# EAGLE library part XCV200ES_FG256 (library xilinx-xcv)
xcv200es_fg256 edit this description Auto generated by make-symbol-device-package-bsdl.ulp Rev. 26 Source: xcv200es_fg256.bsd
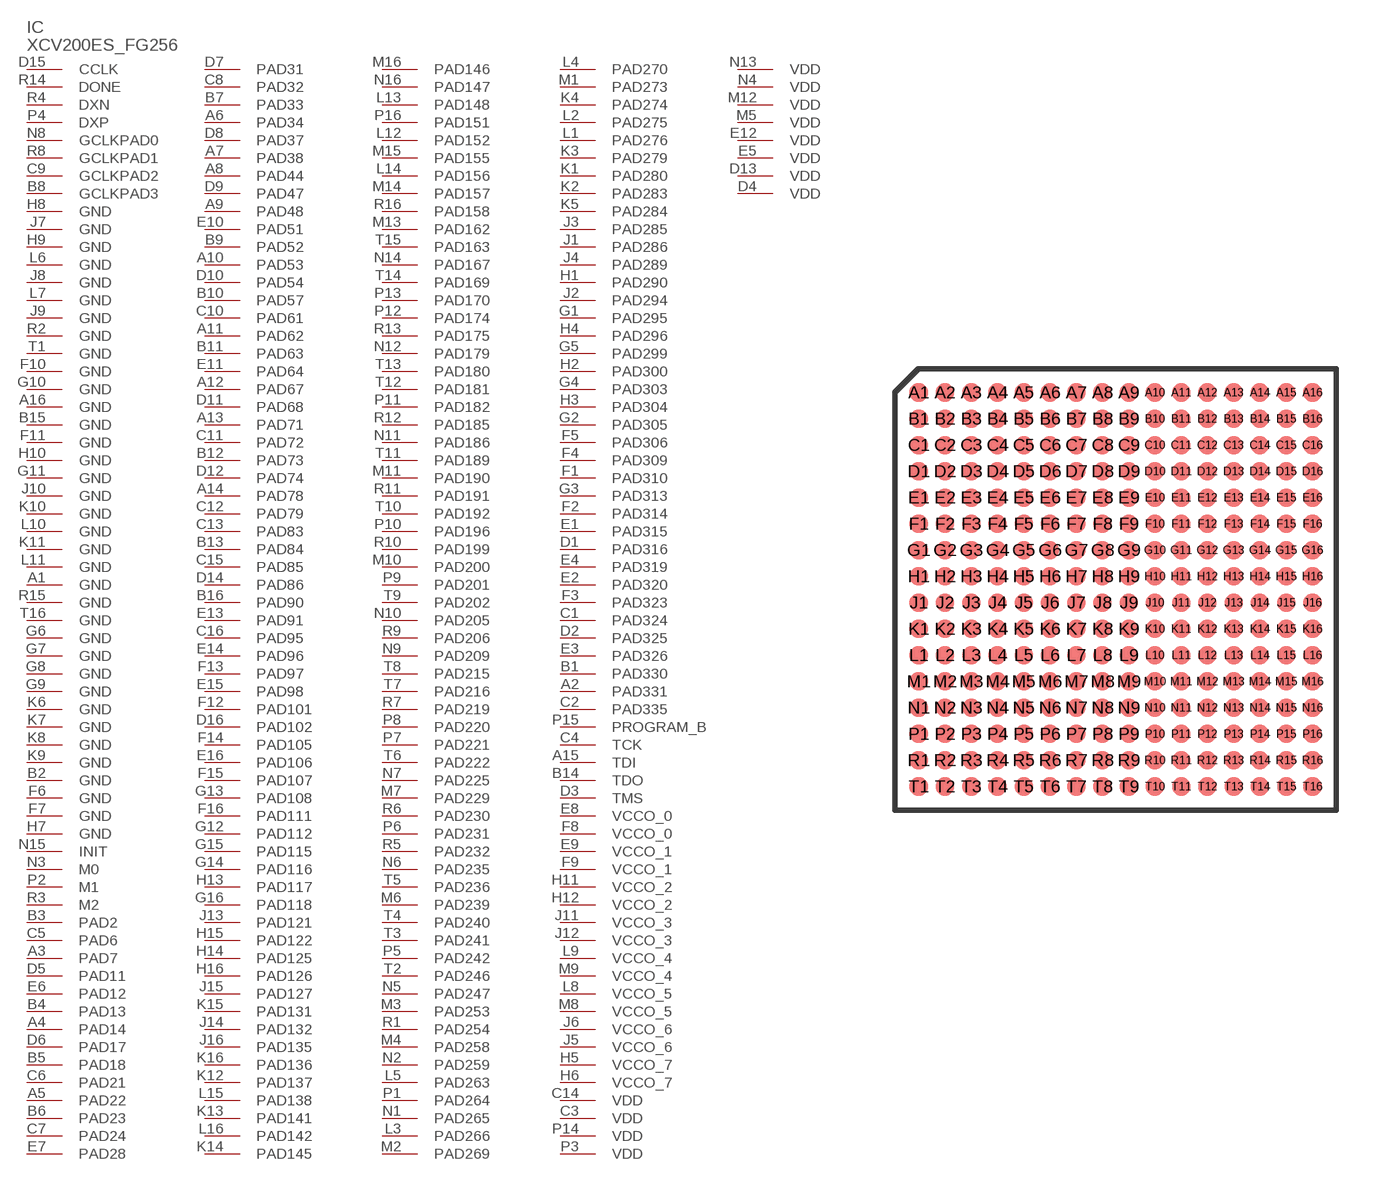
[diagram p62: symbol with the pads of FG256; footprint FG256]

Designator prefix IC

## XCV200ES_FG256 (OC_FARNELL: unknown; OC_NEWARK: unknown)  [FG256]
A1  GND  pwr
A2  PAD331
A3  PAD7
A4  PAD14
A5  PAD22
A6  PAD34
A7  PAD38
A8  PAD44
A9  PAD48
A10  PAD53
A11  PAD62
A12  PAD67
A13  PAD71
A14  PAD78
A15  TDI  in
A16  GND  pwr
B1  PAD330
B2  GND  pwr
B3  PAD2
B4  PAD13
B5  PAD18
B6  PAD23
B7  PAD33
B8  GCLKPAD3  in
B9  PAD52
B10  PAD57
B11  PAD63
B12  PAD73
B13  PAD84
B14  TDO  out
B15  GND  pwr
B16  PAD90
C1  PAD324
C2  PAD335
C3  VDD  pwr
C4  TCK  in
C5  PAD6
C6  PAD21
C7  PAD24
C8  PAD32
C9  GCLKPAD2  in
C10  PAD61
C11  PAD72
C12  PAD79
C13  PAD83
C14  VDD  pwr
C15  PAD85
C16  PAD95
D1  PAD316
D2  PAD325
D3  TMS  in
D4  VDD  pwr
D5  PAD11
D6  PAD17
D7  PAD31
D8  PAD37
D9  PAD47
D10  PAD54
D11  PAD68
D12  PAD74
D13  VDD  pwr
D14  PAD86
D15  CCLK
D16  PAD102
E1  PAD315
E2  PAD320
E3  PAD326
E4  PAD319
E5  VDD  pwr
E6  PAD12
E7  PAD28
E8  VCCO_0  pwr
E9  VCCO_1  pwr
E10  PAD51
E11  PAD64
E12  VDD  pwr
E13  PAD91
E14  PAD96
E15  PAD98
E16  PAD106
F1  PAD310
F2  PAD314
F3  PAD323
F4  PAD309
F5  PAD306
F6  GND  pwr
F7  GND  pwr
F8  VCCO_0  pwr
F9  VCCO_1  pwr
F10  GND  pwr
F11  GND  pwr
F12  PAD101
F13  PAD97
F14  PAD105
F15  PAD107
F16  PAD111
G1  PAD295
G2  PAD305
G3  PAD313
G4  PAD303
G5  PAD299
G6  GND  pwr
G7  GND  pwr
G8  GND  pwr
G9  GND  pwr
G10  GND  pwr
G11  GND  pwr
G12  PAD112
G13  PAD108
G14  PAD116
G15  PAD115
G16  PAD118
H1  PAD290
H2  PAD300
H3  PAD304
H4  PAD296
H5  VCCO_7  pwr
H6  VCCO_7  pwr
H7  GND  pwr
H8  GND  pwr
H9  GND  pwr
H10  GND  pwr
H11  VCCO_2  pwr
H12  VCCO_2  pwr
H13  PAD117
H14  PAD125
H15  PAD122
H16  PAD126
J1  PAD286
J2  PAD294
J3  PAD285
J4  PAD289
J5  VCCO_6  pwr
J6  VCCO_6  pwr
J7  GND  pwr
J8  GND  pwr
J9  GND  pwr
J10  GND  pwr
J11  VCCO_3  pwr
J12  VCCO_3  pwr
J13  PAD121
J14  PAD132
J15  PAD127
J16  PAD135
K1  PAD280
K2  PAD283
K3  PAD279
K4  PAD274
K5  PAD284
K6  GND  pwr
K7  GND  pwr
K8  GND  pwr
K9  GND  pwr
K10  GND  pwr
K11  GND  pwr
K12  PAD137
K13  PAD141
K14  PAD145
K15  PAD131
K16  PAD136
L1  PAD276
L2  PAD275
L3  PAD266
L4  PAD270
L5  PAD263
L6  GND  pwr
L7  GND  pwr
L8  VCCO_5  pwr
L9  VCCO_4  pwr
L10  GND  pwr
L11  GND  pwr
L12  PAD152
L13  PAD148
L14  PAD156
L15  PAD138
L16  PAD142
M1  PAD273
M2  PAD269
M3  PAD253
M4  PAD258
M5  VDD  pwr
M6  PAD239
M7  PAD229
M8  VCCO_5  pwr
M9  VCCO_4  pwr
M10  PAD200
M11  PAD190
M12  VDD  pwr
M13  PAD162
M14  PAD157
M15  PAD155
M16  PAD146
N1  PAD265
N2  PAD259
N3  M0  in
N4  VDD  pwr
N5  PAD247
N6  PAD235
N7  PAD225
N8  GCLKPAD0  in
N9  PAD209
N10  PAD205
N11  PAD186
N12  PAD179
N13  VDD  pwr
N14  PAD167
N15  INIT
N16  PAD147
P1  PAD264
P2  M1  in
P3  VDD  pwr
P4  DXP  pas
P5  PAD242
P6  PAD231
P7  PAD221
P8  PAD220
P9  PAD201
P10  PAD196
P11  PAD182
P12  PAD174
P13  PAD170
P14  VDD  pwr
P15  PROGRAM_B  in
P16  PAD151
R1  PAD254
R2  GND  pwr
R3  M2  in
R4  DXN  pas
R5  PAD232
R6  PAD230
R7  PAD219
R8  GCLKPAD1  in
R9  PAD206
R10  PAD199
R11  PAD191
R12  PAD185
R13  PAD175
R14  DONE
R15  GND  pwr
R16  PAD158
T1  GND  pwr
T2  PAD246
T3  PAD241
T4  PAD240
T5  PAD236
T6  PAD222
T7  PAD216
T8  PAD215
T9  PAD202
T10  PAD192
T11  PAD189
T12  PAD181
T13  PAD180
T14  PAD169
T15  PAD163
T16  GND  pwr

## Footprint FG256 (pad centres in mm)
Fine Pitch BGA (FG256) Auto generated by make-symbol-device-package-bsdl.ulp Rev. 26 Source: xcv100_fg256.bsd; fg256.pdf
smd 0.7 x 0.7: A1 -7.5,7.5; A2 -6.5,7.5; A3 -5.5,7.5; A4 -4.5,7.5; A5 -3.5,7.5; A6 -2.5,7.5; A7 -1.5,7.5; A8 -0.5,7.5; A9 0.5,7.5; A10 1.5,7.5; A11 2.5,7.5; A12 3.5,7.5; A13 4.5,7.5; A14 5.5,7.5; A15 6.5,7.5; A16 7.5,7.5; B1 -7.5,6.5; B2 -6.5,6.5; B3 -5.5,6.5; B4 -4.5,6.5; B5 -3.5,6.5; B6 -2.5,6.5; B7 -1.5,6.5; B8 -0.5,6.5; B9 0.5,6.5; B10 1.5,6.5; B11 2.5,6.5; B12 3.5,6.5; B13 4.5,6.5; B14 5.5,6.5; B15 6.5,6.5; B16 7.5,6.5; C1 -7.5,5.5; C2 -6.5,5.5; C3 -5.5,5.5; C4 -4.5,5.5; C5 -3.5,5.5; C6 -2.5,5.5; C7 -1.5,5.5; C8 -0.5,5.5; C9 0.5,5.5; C10 1.5,5.5; C11 2.5,5.5; C12 3.5,5.5; C13 4.5,5.5; C14 5.5,5.5; C15 6.5,5.5; C16 7.5,5.5; D1 -7.5,4.5; D2 -6.5,4.5; D3 -5.5,4.5; D4 -4.5,4.5; D5 -3.5,4.5; D6 -2.5,4.5; D7 -1.5,4.5; D8 -0.5,4.5; D9 0.5,4.5; D10 1.5,4.5; D11 2.5,4.5; D12 3.5,4.5; D13 4.5,4.5; D14 5.5,4.5; D15 6.5,4.5; D16 7.5,4.5; E1 -7.5,3.5; E2 -6.5,3.5; E3 -5.5,3.5; E4 -4.5,3.5; E5 -3.5,3.5; E6 -2.5,3.5; E7 -1.5,3.5; E8 -0.5,3.5; E9 0.5,3.5; E10 1.5,3.5; E11 2.5,3.5; E12 3.5,3.5; E13 4.5,3.5; E14 5.5,3.5; E15 6.5,3.5; E16 7.5,3.5; F1 -7.5,2.5; F2 -6.5,2.5; F3 -5.5,2.5; F4 -4.5,2.5; F5 -3.5,2.5; F6 -2.5,2.5; F7 -1.5,2.5; F8 -0.5,2.5; F9 0.5,2.5; F10 1.5,2.5; F11 2.5,2.5; F12 3.5,2.5; F13 4.5,2.5; F14 5.5,2.5; F15 6.5,2.5; F16 7.5,2.5; G1 -7.5,1.5; G2 -6.5,1.5; G3 -5.5,1.5; G4 -4.5,1.5; G5 -3.5,1.5; G6 -2.5,1.5; G7 -1.5,1.5; G8 -0.5,1.5; G9 0.5,1.5; G10 1.5,1.5; G11 2.5,1.5; G12 3.5,1.5; G13 4.5,1.5; G14 5.5,1.5; G15 6.5,1.5; G16 7.5,1.5; H1 -7.5,0.5; H2 -6.5,0.5; H3 -5.5,0.5; H4 -4.5,0.5; H5 -3.5,0.5; H6 -2.5,0.5; H7 -1.5,0.5; H8 -0.5,0.5; H9 0.5,0.5; H10 1.5,0.5; H11 2.5,0.5; H12 3.5,0.5; H13 4.5,0.5; H14 5.5,0.5; H15 6.5,0.5; H16 7.5,0.5; J1 -7.5,-0.5; J2 -6.5,-0.5; J3 -5.5,-0.5; J4 -4.5,-0.5; J5 -3.5,-0.5; J6 -2.5,-0.5; J7 -1.5,-0.5; J8 -0.5,-0.5; J9 0.5,-0.5; J10 1.5,-0.5; J11 2.5,-0.5; J12 3.5,-0.5; J13 4.5,-0.5; J14 5.5,-0.5; J15 6.5,-0.5; J16 7.5,-0.5; K1 -7.5,-1.5; K2 -6.5,-1.5; K3 -5.5,-1.5; K4 -4.5,-1.5; K5 -3.5,-1.5; K6 -2.5,-1.5; K7 -1.5,-1.5; K8 -0.5,-1.5; K9 0.5,-1.5; K10 1.5,-1.5; K11 2.5,-1.5; K12 3.5,-1.5; K13 4.5,-1.5; K14 5.5,-1.5; K15 6.5,-1.5; K16 7.5,-1.5; L1 -7.5,-2.5; L2 -6.5,-2.5; L3 -5.5,-2.5; L4 -4.5,-2.5; L5 -3.5,-2.5; L6 -2.5,-2.5; L7 -1.5,-2.5; L8 -0.5,-2.5; L9 0.5,-2.5; L10 1.5,-2.5; L11 2.5,-2.5; L12 3.5,-2.5; L13 4.5,-2.5; L14 5.5,-2.5; L15 6.5,-2.5; L16 7.5,-2.5; M1 -7.5,-3.5; M2 -6.5,-3.5; M3 -5.5,-3.5; M4 -4.5,-3.5; M5 -3.5,-3.5; M6 -2.5,-3.5; M7 -1.5,-3.5; M8 -0.5,-3.5; M9 0.5,-3.5; M10 1.5,-3.5; M11 2.5,-3.5; M12 3.5,-3.5; M13 4.5,-3.5; M14 5.5,-3.5; M15 6.5,-3.5; M16 7.5,-3.5; N1 -7.5,-4.5; N2 -6.5,-4.5; N3 -5.5,-4.5; N4 -4.5,-4.5; N5 -3.5,-4.5; N6 -2.5,-4.5; N7 -1.5,-4.5; N8 -0.5,-4.5; N9 0.5,-4.5; N10 1.5,-4.5; N11 2.5,-4.5; N12 3.5,-4.5; N13 4.5,-4.5; N14 5.5,-4.5; N15 6.5,-4.5; N16 7.5,-4.5; P1 -7.5,-5.5; P2 -6.5,-5.5; P3 -5.5,-5.5; P4 -4.5,-5.5; P5 -3.5,-5.5; P6 -2.5,-5.5; P7 -1.5,-5.5; P8 -0.5,-5.5; P9 0.5,-5.5; P10 1.5,-5.5; P11 2.5,-5.5; P12 3.5,-5.5; P13 4.5,-5.5; P14 5.5,-5.5; P15 6.5,-5.5; P16 7.5,-5.5; R1 -7.5,-6.5; R2 -6.5,-6.5; R3 -5.5,-6.5; R4 -4.5,-6.5; R5 -3.5,-6.5; R6 -2.5,-6.5; R7 -1.5,-6.5; R8 -0.5,-6.5; R9 0.5,-6.5; R10 1.5,-6.5; R11 2.5,-6.5; R12 3.5,-6.5; R13 4.5,-6.5; R14 5.5,-6.5; R15 6.5,-6.5; R16 7.5,-6.5; T1 -7.5,-7.5; T2 -6.5,-7.5; T3 -5.5,-7.5; T4 -4.5,-7.5; T5 -3.5,-7.5; T6 -2.5,-7.5; T7 -1.5,-7.5; T8 -0.5,-7.5; T9 0.5,-7.5; T10 1.5,-7.5; T11 2.5,-7.5; T12 3.5,-7.5; T13 4.5,-7.5; T14 5.5,-7.5; T15 6.5,-7.5; T16 7.5,-7.5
